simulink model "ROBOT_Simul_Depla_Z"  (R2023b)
settings: Solver=ode15s  StartTime=0.0  StopTime=0.2  RelTol=1e-3  EnableMultiTasking=on
undefined symbols (not defined in the file): BATI1_Défaut_sldprt, BATI2_Défaut_sldprt, BATI3_Défaut_sldprt, deg, kg, m, mm, N, rad, s, STL, X, Y, Z
libraries: sm_lib x139, fl_lib x42, nesl_utility x19, slpidlib x3
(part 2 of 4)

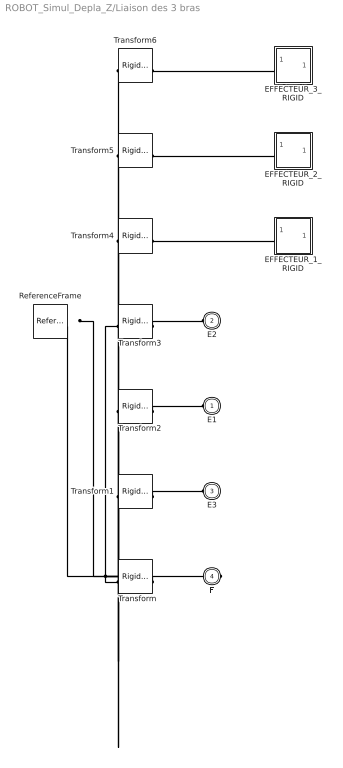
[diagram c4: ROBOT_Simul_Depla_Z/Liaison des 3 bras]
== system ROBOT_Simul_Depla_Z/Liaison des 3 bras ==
  EFFECTEUR_1_RIGID : Subsystem
  EFFECTEUR_2_RIGID : Subsystem
  EFFECTEUR_3_RIGID : Subsystem
  ReferenceFrame : sm_lib/Frames and Transforms/Reference Frame
  Transform : sm_lib/Frames and Transforms/Rigid Transform  TranslationMethod=Cartesian  TranslationStandardOffset=0  TranslationStandardOffsetUnits=mm  TranslationStandardAxis=+Z  TranslationCartesianOffset=[0 0 -32.350000000009082]  TranslationCartesianOffsetUnits=mm  TranslationROffset=0  TranslationROffsetUnits=m  TranslationZOffset=0  TranslationZOffsetUnits=m  TranslationThetaOffset=0  TranslationThetaOffsetUnits=deg  RotationMethod=ArbitraryAxis  RotationAngleUnits=rad  RotationStandardAxis=+Z  RotationAngle=3.1415926535897931  RotationArbitraryAxis=[1 0 0]  FollAlignAxisA=+X  BaseAlignAxisA=+Y  FollAlignAxisB=+Y  BaseAlignAxisB=+Z  RotationSequenceAxes=FollowerAxes  RotationSequence=XYX  RotationSequenceAngles=[0 0 0]  RotationSequenceAnglesUnits=deg  RotationMatrix=[1 0 0; 0 1 0; 0 0 1]  Quaternion=[1 0 0 0]
  Transform1 : sm_lib/Frames and Transforms/Rigid Transform  TranslationMethod=Cartesian  TranslationStandardOffset=0  TranslationStandardOffsetUnits=mm  TranslationStandardAxis=+Z  TranslationCartesianOffset=[-19.120111238677367 -12.995546039657871 14.999999999991132]  TranslationCartesianOffsetUnits=mm  TranslationROffset=0  TranslationROffsetUnits=m  TranslationZOffset=0  TranslationZOffsetUnits=m  TranslationThetaOffset=0  TranslationThetaOffsetUnits=deg  RotationMethod=ArbitraryAxis  RotationAngleUnits=rad  RotationStandardAxis=+Z  RotationAngle=2.4188584057763762  RotationArbitraryAxis=[-0.65465367070797653 -0.37796447300922748 -0.65465367070797764]  FollAlignAxisA=+X  BaseAlignAxisA=+Y  FollAlignAxisB=+Y  BaseAlignAxisB=+Z  RotationSequenceAxes=FollowerAxes  RotationSequence=XYX  RotationSequenceAngles=[0 0 0]  RotationSequenceAnglesUnits=deg  RotationMatrix=[1 0 0; 0 1 0; 0 0 1]  Quaternion=[1 0 0 0]
  Transform2 : sm_lib/Frames and Transforms/Rigid Transform  TranslationMethod=Cartesian  TranslationStandardOffset=0  TranslationStandardOffsetUnits=mm  TranslationStandardAxis=+Z  TranslationCartesianOffset=[2.6286000672859817 43.296105206329507 14.999999999990896]  TranslationCartesianOffsetUnits=mm  TranslationROffset=0  TranslationROffsetUnits=m  TranslationZOffset=0  TranslationZOffsetUnits=m  TranslationThetaOffset=0  TranslationThetaOffsetUnits=deg  RotationMethod=ArbitraryAxis  RotationAngleUnits=rad  RotationStandardAxis=+Z  RotationAngle=2.4188584057763851  RotationArbitraryAxis=[0.65465367070797842 -0.37796447300922287 0.65465367070797842]  FollAlignAxisA=+X  BaseAlignAxisA=+Y  FollAlignAxisB=+Y  BaseAlignAxisB=+Z  RotationSequenceAxes=FollowerAxes  RotationSequence=XYX  RotationSequenceAngles=[0 0 0]  RotationSequenceAnglesUnits=deg  RotationMatrix=[1 0 0; 0 1 0; 0 0 1]  Quaternion=[1 0 0 0]
  Transform3 : sm_lib/Frames and Transforms/Rigid Transform  TranslationMethod=Cartesian  TranslationStandardOffset=0  TranslationStandardOffsetUnits=mm  TranslationStandardAxis=+Z  TranslationCartesianOffset=[43.004244414304381 -8.0147839261255491 14.99999999999091]  TranslationCartesianOffsetUnits=mm  TranslationROffset=0  TranslationROffsetUnits=m  TranslationZOffset=0  TranslationZOffsetUnits=m  TranslationThetaOffset=0  TranslationThetaOffsetUnits=deg  RotationMethod=ArbitraryAxis  RotationAngleUnits=rad  RotationStandardAxis=+Z  RotationAngle=2.0943951023931993  RotationArbitraryAxis=[-0.57735026918962318 -0.57735026918962706 0.57735026918962695]  FollAlignAxisA=+X  BaseAlignAxisA=+Y  FollAlignAxisB=+Y  BaseAlignAxisB=+Z  RotationSequenceAxes=FollowerAxes  RotationSequence=XYX  RotationSequenceAngles=[0 0 0]  RotationSequenceAnglesUnits=deg  RotationMatrix=[1 0 0; 0 1 0; 0 0 1]  Quaternion=[1 0 0 0]
  Transform4 : sm_lib/Frames and Transforms/Rigid Transform  TranslationMethod=Cartesian  TranslationStandardOffset=0  TranslationStandardOffsetUnits=mm  TranslationStandardAxis=+Z  TranslationCartesianOffset=[8.0042444143042797 5.9852160738742057 -9.0899510141184692e-12]  TranslationCartesianOffsetUnits=mm  TranslationROffset=0  TranslationROffsetUnits=m  TranslationZOffset=0  TranslationZOffsetUnits=m  TranslationThetaOffset=0  TranslationThetaOffsetUnits=deg  RotationMethod=None  RotationAngleUnits=deg  RotationStandardAxis=+Z  RotationAngle=0  RotationArbitraryAxis=[0 0 1]  FollAlignAxisA=+X  BaseAlignAxisA=+Y  FollAlignAxisB=+Y  BaseAlignAxisB=+Z  RotationSequenceAxes=FollowerAxes  RotationSequence=XYX  RotationSequenceAngles=[0 0 0]  RotationSequenceAnglesUnits=deg  RotationMatrix=[1 0 0; 0 1 0; 0 0 1]  Quaternion=[1 0 0 0]
  Transform5 : sm_lib/Frames and Transforms/Rigid Transform  TranslationMethod=Cartesian  TranslationStandardOffset=0  TranslationStandardOffsetUnits=mm  TranslationStandardAxis=+Z  TranslationCartesianOffset=[8.0042444143042797 5.9852160738742057 -9.0899510141184692e-12]  TranslationCartesianOffsetUnits=mm  TranslationROffset=0  TranslationROffsetUnits=m  TranslationZOffset=0  TranslationZOffsetUnits=m  TranslationThetaOffset=0  TranslationThetaOffsetUnits=deg  RotationMethod=ArbitraryAxis  RotationAngleUnits=rad  RotationStandardAxis=+Z  RotationAngle=2.0943951023932001  RotationArbitraryAxis=[0 0 1]  FollAlignAxisA=+X  BaseAlignAxisA=+Y  FollAlignAxisB=+Y  BaseAlignAxisB=+Z  RotationSequenceAxes=FollowerAxes  RotationSequence=XYX  RotationSequenceAngles=[0 0 0]  RotationSequenceAnglesUnits=deg  RotationMatrix=[1 0 0; 0 1 0; 0 0 1]  Quaternion=[1 0 0 0]
  Transform6 : sm_lib/Frames and Transforms/Rigid Transform  TranslationMethod=Cartesian  TranslationStandardOffset=0  TranslationStandardOffsetUnits=mm  TranslationStandardAxis=+Z  TranslationCartesianOffset=[8.0042444143042797 5.9852160738742057 -9.0899510141184692e-12]  TranslationCartesianOffsetUnits=mm  TranslationROffset=0  TranslationROffsetUnits=m  TranslationZOffset=0  TranslationZOffsetUnits=m  TranslationThetaOffset=0  TranslationThetaOffsetUnits=deg  RotationMethod=ArbitraryAxis  RotationAngleUnits=rad  RotationStandardAxis=+Z  RotationAngle=2.0943951023931859  RotationArbitraryAxis=[-0 -0 -1]  FollAlignAxisA=+X  BaseAlignAxisA=+Y  FollAlignAxisB=+Y  BaseAlignAxisB=+Z  RotationSequenceAxes=FollowerAxes  RotationSequence=XYX  RotationSequenceAngles=[0 0 0]  RotationSequenceAnglesUnits=deg  RotationMatrix=[1 0 0; 0 1 0; 0 0 1]  Quaternion=[1 0 0 0]
  E1 : PMIOPort  Side=Left
  E2 : PMIOPort  Port=2  Side=Left
  E3 : PMIOPort  Port=3  Side=Left
  F : PMIOPort  Port=4  Side=Right
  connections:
  Transform/LConn1 -- ReferenceFrame/RConn1 -- Transform1/LConn1 -- Transform2/LConn1 -- Transform3/LConn1 -- Transform4/LConn1 -- Transform5/LConn1 -- Transform6/LConn1
  Transform/RConn1 -- F/RConn1
  Transform1/RConn1 -- E3/RConn1
  Transform2/RConn1 -- E1/RConn1
  Transform3/RConn1 -- E2/RConn1
  EFFECTEUR_1_RIGID/LConn1 -- Transform4/RConn1
  EFFECTEUR_2_RIGID/LConn1 -- Transform5/RConn1
  EFFECTEUR_3_RIGID/LConn1 -- Transform6/RConn1

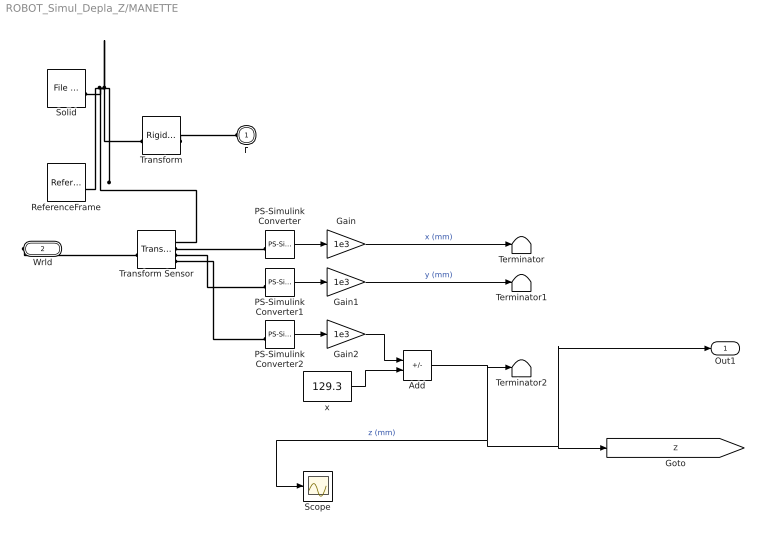
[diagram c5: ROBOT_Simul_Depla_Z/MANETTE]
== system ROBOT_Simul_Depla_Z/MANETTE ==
  Add : Sum  Inputs=+-
  Gain : Gain  Gain=1e3
  Gain1 : Gain  Gain=1e3
  Gain2 : Gain  Gain=1e3
  PS-Simulink Converter : nesl_utility/PS-Simulink Converter  PhysicalDomain=network_engine_domain  SubClassName=ps_output  LeftPortType=input  RightPortType=output  PseudoPeriodic=off  Frequencies=[]  VectorFormat=1-D array  Unit=1  AffineConversion=off
  PS-Simulink Converter1 : nesl_utility/PS-Simulink Converter  PhysicalDomain=network_engine_domain  SubClassName=ps_output  LeftPortType=input  RightPortType=output  PseudoPeriodic=off  Frequencies=[]  VectorFormat=1-D array  Unit=1  AffineConversion=off
  PS-Simulink Converter2 : nesl_utility/PS-Simulink Converter  PhysicalDomain=network_engine_domain  SubClassName=ps_output  LeftPortType=input  RightPortType=output  PseudoPeriodic=off  Frequencies=[]  VectorFormat=1-D array  Unit=1  AffineConversion=off
  ReferenceFrame : sm_lib/Frames and Transforms/Reference Frame
  Scope : Scope
  Solid : sm_lib/Body Elements/File Solid  ExtGeomFileName=\STL\MANETTE_Défaut_sldprt.STL  UnitType=Custom  ExtGeomFileUnits=mm  StepReaderType=HEX  ExportConvexHullGeometry=off  InertiaType=Custom  Mass=0.040615337241087436  MassUnits=kg  CenterOfMass=[0 0.040047984959972249 0]  CenterOfMassUnits=mm  MomentsOfInertia=[8.2576276174464649 8.2126567442848692 8.2576263457676724]  MomentsOfInertiaUnits=kg*mm^2  ProductsOfInertia=[0 0 0]  ProductsOfInertiaUnits=kg*mm^2  BasedOnType=Density  Density=1000  DensityUnits=kg/(m^3)  DoExposeReferenceFrame=on  SerializedFrames=<Frames/>  GraphicType=FromGeometry  MarkerShape=Sphere  MarkerSize=10  MarkerSizeUnits=m  GraphicVisPropType=SimpleVisualProperties  GraphicDiffuseColor=[0.69803921568627447 0.69803921568627447 0.69803921568627447]  GraphicSpecularColor=[0.5 0.5 0.5 1.0]  GraphicAmbientColor=[0.15 0.15 0.15 1.0]  GraphicEmissiveColor=[0.0 0.0 0.0 1.0]  GraphicShininess=75  GraphicOpacity=1
  Terminator : Terminator
  Terminator1 : Terminator
  Terminator2 : Terminator
  Transform : sm_lib/Frames and Transforms/Rigid Transform  TranslationMethod=Cartesian  TranslationStandardOffset=0  TranslationStandardOffsetUnits=mm  TranslationStandardAxis=+Z  TranslationCartesianOffset=[-8.0042444143042815 2.4868995751603507e-14 5.9852160738742031]  TranslationCartesianOffsetUnits=mm  TranslationROffset=0  TranslationROffsetUnits=m  TranslationZOffset=0  TranslationZOffsetUnits=m  TranslationThetaOffset=0  TranslationThetaOffsetUnits=deg  RotationMethod=ArbitraryAxis  RotationAngleUnits=rad  RotationStandardAxis=+Z  RotationAngle=1.570796326794897  RotationArbitraryAxis=[1 -1.5700924586837747e-16 -7.5435830438090697e-17]  FollAlignAxisA=+X  BaseAlignAxisA=+Y  FollAlignAxisB=+Y  BaseAlignAxisB=+Z  RotationSequenceAxes=FollowerAxes  RotationSequence=XYX  RotationSequenceAngles=[0 0 0]  RotationSequenceAnglesUnits=deg  RotationMatrix=[1 0 0; 0 1 0; 0 0 1]  Quaternion=[1 0 0 0]
  Transform Sensor : sm_lib/Frames and Transforms/Transform Sensor  MeasurementFrame=World  RotationSequence=XYX  SenseAngle=off  SenseAxis=off  SenseQ=off  SenseR=off  SenseRotationSequence=off  SenseOmegaX=off  SenseOmegaY=off  SenseOmegaZ=off  SenseOmega=off  SenseQDot=off  SenseRDot=off  SenseRotationSequenceDot=off  SenseAlphaX=off  SenseAlphaY=off  SenseAlphaZ=off  SenseAlpha=off  SenseQDDot=off  SenseRDDot=off  SenseX=on  SenseY=on  SenseZ=on  SenseXYZ=off  SenseRad=off  SenseAzim=off  SenseDist=off  SenseInc=off  SenseXDot=off  SenseYDot=off  SenseZDot=off  SenseXYZDot=off  SenseRadDot=off  SenseAzimDot=off  SenseDistDot=off  SenseIncDot=off  SenseXDDot=off  SenseYDDot=off  SenseZDDot=off  SenseXYZDDot=off  SenseRadDDot=off  SenseAzimDDot=off  SenseDistDDot=off  SenseIncDDot=off
  x : Constant  Value=129.3
  F : PMIOPort  Side=Left
  Wrld : PMIOPort  Port=2  Side=Right
  Out1 : Outport  VectorParamsAs1DForOutWhenUnconnected=off
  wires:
  Gain1/1 -> Terminator1/1  "y (mm)"
  PS-Simulink Converter2/1 -> Gain2/1
  x/1 -> Add/2
  Add/1 -> Scope/1, Out1/1, [Z], Terminator2/1  "z (mm)"
  PS-Simulink Converter1/1 -> Gain1/1
  Gain2/1 -> Add/1
  PS-Simulink Converter/1 -> Gain/1
  Gain/1 -> Terminator/1  "x (mm)"
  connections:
  Solid/RConn1 -- ReferenceFrame/RConn1 -- Transform Sensor/RConn1 -- Transform/LConn1
  Transform/RConn1 -- F/RConn1
  PS-Simulink Converter2/LConn1 -- Transform Sensor/RConn4
  Transform Sensor/RConn3 -- PS-Simulink Converter1/LConn1
  Transform Sensor/RConn2 -- PS-Simulink Converter/LConn1
  Wrld/RConn1 -- Transform Sensor/LConn1

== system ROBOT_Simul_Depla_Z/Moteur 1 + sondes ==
  In1 : Inport
  Moteur à courant continu1 : Subsystem
  Reference electrique : fl_lib/Electrical/Electrical Elements/Electrical Reference
  Simulink-PS Converter1 : nesl_utility/Simulink-PS Converter  PhysicalDomain=network_engine_domain  SubClassName=ps_input  LeftPortType=input  RightPortType=output  PseudoPeriodic=off  Frequencies=[]  NoiseDistribution=none  NoiseParameters=[]  Unit=V  AffineConversion=off  FilteringAndDerivatives=zero  SimscapeFilterOrder=2  InputFilterTimeConstant=1e-4  UdotUserProvided=1
  Sondes électriques1 : Subsystem
  Source de tension controlée1 : fl_lib/Electrical/Electrical Sources/Controlled Voltage Source
  Conn1 : PMIOPort  Side=Right
  Conn2 : PMIOPort  Port=2  Side=Right
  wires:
  In1/1 -> Simulink-PS Converter1/1
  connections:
  Conn2/RConn1 -- Moteur à courant continu1/RConn2
  Conn1/RConn1 -- Moteur à courant continu1/RConn1
  Source de tension controlée1/LConn1 -- Sondes électriques1/LConn1
  Simulink-PS Converter1/RConn1 -- Source de tension controlée1/RConn1
  Sondes électriques1/RConn2 -- Source de tension controlée1/RConn2 -- Reference electrique/LConn1 -- Moteur à courant continu1/LConn2
  Sondes électriques1/RConn1 -- Moteur à courant continu1/LConn1

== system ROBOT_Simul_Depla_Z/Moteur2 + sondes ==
  In1 : Inport
  Moteur à courant continu2 : Subsystem
  Reference electrique : fl_lib/Electrical/Electrical Elements/Electrical Reference
  Simulink-PS Converter1 : nesl_utility/Simulink-PS Converter  PhysicalDomain=network_engine_domain  SubClassName=ps_input  LeftPortType=input  RightPortType=output  PseudoPeriodic=off  Frequencies=[]  NoiseDistribution=none  NoiseParameters=[]  Unit=V  AffineConversion=off  FilteringAndDerivatives=zero  SimscapeFilterOrder=2  InputFilterTimeConstant=1e-4  UdotUserProvided=1
  Sondes électriques : Subsystem
  Source de tension controlée : fl_lib/Electrical/Electrical Sources/Controlled Voltage Source
  Conn1 : PMIOPort  Side=Right
  Conn2 : PMIOPort  Port=2  Side=Right
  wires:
  In1/1 -> Simulink-PS Converter1/1
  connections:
  Sondes électriques/RConn1 -- Moteur à courant continu2/LConn1
  Source de tension controlée/RConn2 -- Reference electrique/LConn1 -- Sondes électriques/RConn2 -- Moteur à courant continu2/LConn2
  Simulink-PS Converter1/RConn1 -- Source de tension controlée/RConn1
  Source de tension controlée/LConn1 -- Sondes électriques/LConn1
  Conn1/RConn1 -- Moteur à courant continu2/RConn1
  Conn2/RConn1 -- Moteur à courant continu2/RConn2

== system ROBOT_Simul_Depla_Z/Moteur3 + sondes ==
  In1 : Inport
  Moteur à courant continu3 : Subsystem
  Reference electrique : fl_lib/Electrical/Electrical Elements/Electrical Reference
  Simulink-PS Converter1 : nesl_utility/Simulink-PS Converter  PhysicalDomain=network_engine_domain  SubClassName=ps_input  LeftPortType=input  RightPortType=output  PseudoPeriodic=off  Frequencies=[]  NoiseDistribution=none  NoiseParameters=[]  Unit=V  AffineConversion=off  FilteringAndDerivatives=zero  SimscapeFilterOrder=2  InputFilterTimeConstant=1e-4  UdotUserProvided=1
  Sondes électriques3 : Subsystem
  Source de tension controlée3 : fl_lib/Electrical/Electrical Sources/Controlled Voltage Source
  Conn1 : PMIOPort  Side=Right
  Conn2 : PMIOPort  Port=2  Side=Right
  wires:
  In1/1 -> Simulink-PS Converter1/1
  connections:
  Sondes électriques3/RConn1 -- Moteur à courant continu3/LConn1
  Moteur à courant continu3/LConn2 -- Reference electrique/LConn1 -- Source de tension controlée3/RConn2 -- Sondes électriques3/RConn2
  Simulink-PS Converter1/RConn1 -- Source de tension controlée3/RConn1
  Source de tension controlée3/LConn1 -- Sondes électriques3/LConn1
  Conn1/RConn1 -- Moteur à courant continu3/RConn1
  Conn2/RConn1 -- Moteur à courant continu3/RConn2

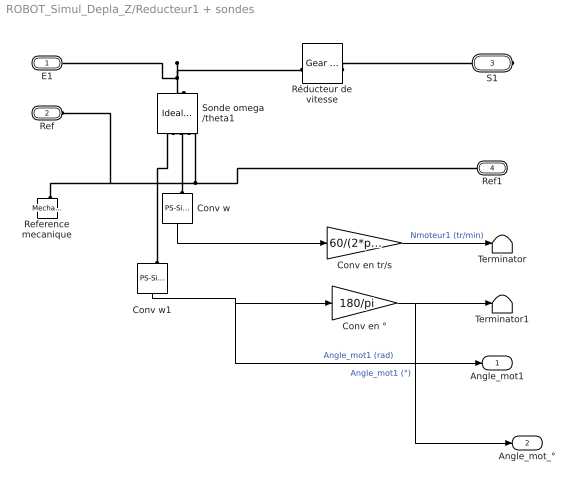
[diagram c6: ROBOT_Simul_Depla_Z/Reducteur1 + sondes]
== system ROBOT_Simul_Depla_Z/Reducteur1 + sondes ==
  Conv en tr/s : Gain  Gain=60/(2*pi)
  Conv en ° : Gain  Gain=180/pi
  Conv w : nesl_utility/PS-Simulink Converter  PhysicalDomain=network_engine_domain  SubClassName=ps_output  LeftPortType=input  RightPortType=output  PseudoPeriodic=off  Frequencies=[]  VectorFormat=1-D array  Unit=1  AffineConversion=off
  Conv w1 : nesl_utility/PS-Simulink Converter  PhysicalDomain=network_engine_domain  SubClassName=ps_output  LeftPortType=input  RightPortType=output  PseudoPeriodic=off  Frequencies=[]  VectorFormat=1-D array  Unit=1  AffineConversion=off
  Reference mecanique : fl_lib/Mechanical/Rotational Elements/Mechanical Rotational Reference
  Réducteur de vitesse : fl_lib/Mechanical/Mechanisms/Gear Box  ratio=7.627  t_in_specify=off  t_in_priority=None  t_in=0 N*m  t_in_nominal_specify=off  t_in_nominal_unit=N*m  t_in_nominal_value=1  t_out_specify=off  t_out_priority=None  t_out=0 N*m  t_out_nominal_specify=off  t_out_nominal_unit=N*m  t_out_nominal_value=1
  Sonde omega /theta1 : fl_lib/Mechanical/Mechanical Sensors/Ideal Rotational Motion Sensor  reference=foundation.enum.MeasurementReference.difference  acceleration_port=false  velocity_port=true  position_port=true  wrap_angle=false  offset=0 rad
  Terminator : Terminator
  Terminator1 : Terminator
  E1 : PMIOPort  Side=Left
  Ref : PMIOPort  Port=2  Side=Left
  S1 : PMIOPort  Port=3  Side=Right
  Ref1 : PMIOPort  Port=4  Side=Right
  Angle_mot1 : Outport  VectorParamsAs1DForOutWhenUnconnected=off
  Angle_mot_° : Outport  Port=2  VectorParamsAs1DForOutWhenUnconnected=off
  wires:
  Conv w1/1 -> Angle_mot1/1, Conv en °/1  "Angle_mot1 (rad)"
  Conv en °/1 -> Angle_mot_°/1, Terminator1/1  "Angle_mot1 (°)"
  Conv w/1 -> Conv en tr/s/1
  Conv en tr/s/1 -> Terminator/1  "Nmoteur1 (tr/min)"
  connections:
  Sonde omega /theta1/LConn1 -- E1/RConn1 -- Réducteur de vitesse/LConn1
  Reference mecanique/LConn1 -- Ref/RConn1 -- Sonde omega /theta1/RConn1 -- Ref1/RConn1
  Conv w/LConn1 -- Sonde omega /theta1/RConn2
  Conv w1/LConn1 -- Sonde omega /theta1/RConn3
  Réducteur de vitesse/RConn1 -- S1/RConn1

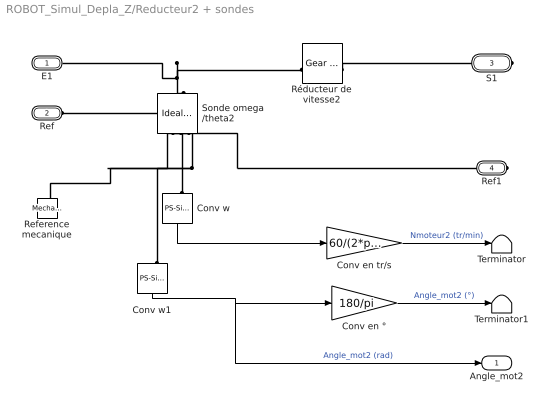
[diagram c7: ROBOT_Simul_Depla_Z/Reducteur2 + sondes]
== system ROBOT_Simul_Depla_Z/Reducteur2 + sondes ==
  Conv en tr/s : Gain  Gain=60/(2*pi)
  Conv en ° : Gain  Gain=180/pi
  Conv w : nesl_utility/PS-Simulink Converter  PhysicalDomain=network_engine_domain  SubClassName=ps_output  LeftPortType=input  RightPortType=output  PseudoPeriodic=off  Frequencies=[]  VectorFormat=1-D array  Unit=1  AffineConversion=off
  Conv w1 : nesl_utility/PS-Simulink Converter  PhysicalDomain=network_engine_domain  SubClassName=ps_output  LeftPortType=input  RightPortType=output  PseudoPeriodic=off  Frequencies=[]  VectorFormat=1-D array  Unit=1  AffineConversion=off
  Reference mecanique : fl_lib/Mechanical/Rotational Elements/Mechanical Rotational Reference
  Réducteur de vitesse2 : fl_lib/Mechanical/Mechanisms/Gear Box  ratio=7.627  t_in_specify=off  t_in_priority=None  t_in=0 N*m  t_in_nominal_specify=off  t_in_nominal_unit=N*m  t_in_nominal_value=1  t_out_specify=off  t_out_priority=None  t_out=0 N*m  t_out_nominal_specify=off  t_out_nominal_unit=N*m  t_out_nominal_value=1
  Sonde omega /theta2 : fl_lib/Mechanical/Mechanical Sensors/Ideal Rotational Motion Sensor  reference=foundation.enum.MeasurementReference.difference  acceleration_port=false  velocity_port=true  position_port=true  wrap_angle=false  offset=0 rad
  Terminator : Terminator
  Terminator1 : Terminator
  E1 : PMIOPort  Side=Left
  Ref : PMIOPort  Port=2  Side=Left
  S1 : PMIOPort  Port=3  Side=Right
  Ref1 : PMIOPort  Port=4  Side=Right
  Angle_mot2 : Outport  VectorParamsAs1DForOutWhenUnconnected=off
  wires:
  Conv w1/1 -> Angle_mot2/1, Conv en °/1  "Angle_mot2 (rad)"
  Conv en °/1 -> Terminator1/1  "Angle_mot2 (°)"
  Conv w/1 -> Conv en tr/s/1
  Conv en tr/s/1 -> Terminator/1  "Nmoteur2 (tr/min)"
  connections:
  Sonde omega /theta2/LConn1 -- E1/RConn1 -- Réducteur de vitesse2/LConn1
  Ref1/RConn1 -- Sonde omega /theta2/RConn1 -- Reference mecanique/LConn1 -- Ref/RConn1
  Conv w1/LConn1 -- Sonde omega /theta2/RConn3
  Conv w/LConn1 -- Sonde omega /theta2/RConn2
  Réducteur de vitesse2/RConn1 -- S1/RConn1

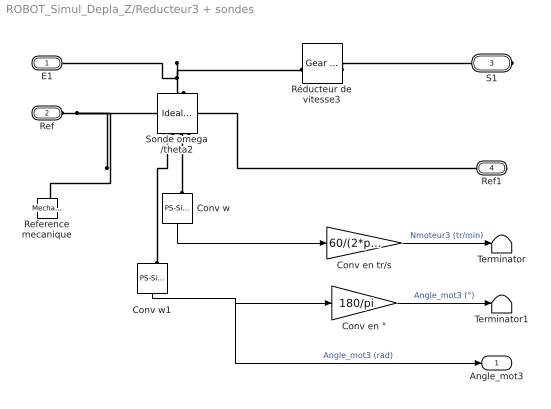
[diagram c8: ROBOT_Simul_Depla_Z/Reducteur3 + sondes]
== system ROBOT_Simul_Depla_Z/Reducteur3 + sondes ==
  Conv en tr/s : Gain  Gain=60/(2*pi)
  Conv en ° : Gain  Gain=180/pi
  Conv w : nesl_utility/PS-Simulink Converter  PhysicalDomain=network_engine_domain  SubClassName=ps_output  LeftPortType=input  RightPortType=output  PseudoPeriodic=off  Frequencies=[]  VectorFormat=1-D array  Unit=1  AffineConversion=off
  Conv w1 : nesl_utility/PS-Simulink Converter  PhysicalDomain=network_engine_domain  SubClassName=ps_output  LeftPortType=input  RightPortType=output  PseudoPeriodic=off  Frequencies=[]  VectorFormat=1-D array  Unit=1  AffineConversion=off
  Reference mecanique : fl_lib/Mechanical/Rotational Elements/Mechanical Rotational Reference
  Réducteur de vitesse3 : fl_lib/Mechanical/Mechanisms/Gear Box  ratio=-7.627  t_in_specify=off  t_in_priority=None  t_in=0 N*m  t_in_nominal_specify=off  t_in_nominal_unit=N*m  t_in_nominal_value=1  t_out_specify=off  t_out_priority=None  t_out=0 N*m  t_out_nominal_specify=off  t_out_nominal_unit=N*m  t_out_nominal_value=1
  Sonde omega /theta2 : fl_lib/Mechanical/Mechanical Sensors/Ideal Rotational Motion Sensor  reference=foundation.enum.MeasurementReference.difference  acceleration_port=false  velocity_port=true  position_port=true  wrap_angle=false  offset=0 rad
  Terminator : Terminator
  Terminator1 : Terminator
  E1 : PMIOPort  Side=Left
  Ref : PMIOPort  Port=2  Side=Left
  S1 : PMIOPort  Port=3  Side=Right
  Ref1 : PMIOPort  Port=4  Side=Right
  Angle_mot3 : Outport  VectorParamsAs1DForOutWhenUnconnected=off
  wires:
  Conv w1/1 -> Angle_mot3/1, Conv en °/1  "Angle_mot3 (rad)"
  Conv en °/1 -> Terminator1/1  "Angle_mot3 (°)"
  Conv w/1 -> Conv en tr/s/1
  Conv en tr/s/1 -> Terminator/1  "Nmoteur3 (tr/min)"
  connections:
  Sonde omega /theta2/LConn1 -- E1/RConn1 -- Réducteur de vitesse3/LConn1
  Ref/RConn1 -- Reference mecanique/LConn1 -- Sonde omega /theta2/RConn1 -- Ref1/RConn1
  Conv w1/LConn1 -- Sonde omega /theta2/RConn3
  Réducteur de vitesse3/RConn1 -- S1/RConn1
  Conv w/LConn1 -- Sonde omega /theta2/RConn2

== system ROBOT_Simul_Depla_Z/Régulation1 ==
  In1 : Inport
  In2 : Inport  Port=2
  Add : Sum  Inputs=-+
  PID Controller : slpidlib/PID Controller  Controller=PD  Form=Parallel  TimeDomain=Continuous-time  UseExternalTs=off  SampleTime=1  IntegratorMethod=Forward Euler  FilterMethod=Forward Euler  ControllerParametersSource=internal  P=200  I=30  UseKiTs=off  D=4  N=900  UseFilter=on  TunerSelectOption=Transfer Function Based (PID Tuner App)  ZeroCross=off  InitialConditionSource=internal  InitialConditionForIntegrator=0  InitialConditionForFilter=0  DifferentiatorICPrevScaledInput=0  ExternalReset=none  TrackingMode=off  Kt=1  LimitOutput=on  SatLimitsSource=internal  UpperSaturationLimit=30  LowerSaturationLimit=-30  LinearizeAsGain=off  AntiWindupMode=none  Kb=1  LimitIntegrator=off  UpperIntegratorSaturationLimit=inf  LowerIntegratorSaturationLimit=-inf  POutMin=[]  POutMax=[]  IOutMin=[]  IOutMax=[]  DOutMin=[]  DOutMax=[]  NOutMin=[]  NOutMax=[]  SumOutMin=[]  SumOutMax=[]  SaturationOutMin=[]  SaturationOutMax=[]  PParamMin=[]  PParamMax=[]  IParamMin=[]  IParamMax=[]  DParamMin=[]  DParamMax=[]  NParamMin=[]  NParamMax=[]  KbParamMin=[]  KbParamMax=[]  KtParamMin=[]  KtParamMax=[]  KbOutMin=[]  KbOutMax=[]  KtOutMin=[]  KtOutMax=[]  IntegratorOutMin=[]  IntegratorOutMax=[]  FilterOutMin=[]  FilterOutMax=[]  SumI1OutMin=[]  SumI1OutMax=[]  SumI2OutMin=[]  SumI2OutMax=[]  SumI3OutMin=[]  SumI3OutMax=[]  SumI4OutMin=[]  SumI4OutMax=[]  SumDOutMin=[]  SumDOutMax=[]  DifferentiatorOutMin=[]  DifferentiatorOutMax=[]  FilterDiffOutCoefMin=[]  FilterDiffOutCoefMax=[]  ReciprocalOutMin=[]  ReciprocalOutMax=[]  SumDenOutMin=[]  SumDenOutMax=[]  SumNumOutMin=[]  SumNumOutMax=[]  DivideOutMin=[]  DivideOutMax=[]  UdiffTsProdOutMin=[]  UdiffTsProdOutMax=[]  NTsProdOutMin=[]  NTsProdOutMax=[]  UintegralTsProdOutMin=[]  UintegralTsProdOutMax=[]  UngainTsProdOutMin=[]  UngainTsProdOutMax=[]  ClampingZeroOutDataTypeStr=Inherit: Inherit via back propagation  ClampingZeroOutMin=[]  ClampingZeroOutMax=[]  FilterDenConstantOutDataTypeStr=Inherit: Inherit via back propagation  FilterDenConstantOutMin=[]  FilterDenConstantOutMax=[]  PCopyOutDataTypeStr=Inherit: Inherit via back propagation  PCopyOutMin=[]  PCopyOutMax=[]  NCopyOutDataTypeStr=Inherit: Inherit via back propagation  NCopyOutMin=[]  NCopyOutMax=[]  IntegratorContinuousStateAttributes=''  IntegratorStateMustResolveToSignalObject=off  IntegratorRTWStateStorageClass=Auto  FilterContinuousStateAttributes=''  FilterStateMustResolveToSignalObject=off  FilterRTWStateStorageClass=Auto  ParallelPVariant=InternalParameters  IdealPVariant=Disabled  IVariant=Disabled  DVariant=InternalParameters  IntegratorVariant=Disabled  SatVariant=Enabled  AWVariant=Disabled  PCopyVariant=Disabled  TRVariant=Disabled  FdbkBlocksVariant=Forward  IdealPFdbkVariant=Disabled  SatFdbkVariant=Disabled  DerivativeFilterVariant=ContFilter  NVariant=InternalParameters  NCopyVariant=Disabled  FilterICVariant=InternalICsFilter  IntegratorICVariant=Disabled  ExternalResetVariant=Disabled  TRSumVariant=Passthrough  SumFdbkVariant=Disabled  SumVariant=Sum_PD  TsampFilterVariant=InternalTs  TsampNgainVariant=Passthrough  TsampIntegralVariant=Disabled_SignalSpec  ExternalSaturationOutDataTypeStr=Inherit: Same as second input
  Out1 : Outport  VectorParamsAs1DForOutWhenUnconnected=off
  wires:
  In1/1 -> Add/1
  In2/1 -> Add/2
  PID Controller/1 -> Out1/1
  Add/1 -> PID Controller/1

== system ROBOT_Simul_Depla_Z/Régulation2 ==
  In1 : Inport
  In2 : Inport  Port=2
  Add : Sum  Inputs=-+
  PID Controller : slpidlib/PID Controller  Controller=PD  Form=Parallel  TimeDomain=Continuous-time  UseExternalTs=off  SampleTime=1  IntegratorMethod=Forward Euler  FilterMethod=Forward Euler  ControllerParametersSource=internal  P=200  I=30  UseKiTs=off  D=4  N=900  UseFilter=on  TunerSelectOption=Transfer Function Based (PID Tuner App)  ZeroCross=off  InitialConditionSource=internal  InitialConditionForIntegrator=0  InitialConditionForFilter=0  DifferentiatorICPrevScaledInput=0  ExternalReset=none  TrackingMode=off  Kt=1  LimitOutput=on  SatLimitsSource=internal  UpperSaturationLimit=30  LowerSaturationLimit=-30  LinearizeAsGain=off  AntiWindupMode=none  Kb=1  LimitIntegrator=off  UpperIntegratorSaturationLimit=inf  LowerIntegratorSaturationLimit=-inf  POutMin=[]  POutMax=[]  IOutMin=[]  IOutMax=[]  DOutMin=[]  DOutMax=[]  NOutMin=[]  NOutMax=[]  SumOutMin=[]  SumOutMax=[]  SaturationOutMin=[]  SaturationOutMax=[]  PParamMin=[]  PParamMax=[]  IParamMin=[]  IParamMax=[]  DParamMin=[]  DParamMax=[]  NParamMin=[]  NParamMax=[]  KbParamMin=[]  KbParamMax=[]  KtParamMin=[]  KtParamMax=[]  KbOutMin=[]  KbOutMax=[]  KtOutMin=[]  KtOutMax=[]  IntegratorOutMin=[]  IntegratorOutMax=[]  FilterOutMin=[]  FilterOutMax=[]  SumI1OutMin=[]  SumI1OutMax=[]  SumI2OutMin=[]  SumI2OutMax=[]  SumI3OutMin=[]  SumI3OutMax=[]  SumI4OutMin=[]  SumI4OutMax=[]  SumDOutMin=[]  SumDOutMax=[]  DifferentiatorOutMin=[]  DifferentiatorOutMax=[]  FilterDiffOutCoefMin=[]  FilterDiffOutCoefMax=[]  ReciprocalOutMin=[]  ReciprocalOutMax=[]  SumDenOutMin=[]  SumDenOutMax=[]  SumNumOutMin=[]  SumNumOutMax=[]  DivideOutMin=[]  DivideOutMax=[]  UdiffTsProdOutMin=[]  UdiffTsProdOutMax=[]  NTsProdOutMin=[]  NTsProdOutMax=[]  UintegralTsProdOutMin=[]  UintegralTsProdOutMax=[]  UngainTsProdOutMin=[]  UngainTsProdOutMax=[]  ClampingZeroOutDataTypeStr=Inherit: Inherit via back propagation  ClampingZeroOutMin=[]  ClampingZeroOutMax=[]  FilterDenConstantOutDataTypeStr=Inherit: Inherit via back propagation  FilterDenConstantOutMin=[]  FilterDenConstantOutMax=[]  PCopyOutDataTypeStr=Inherit: Inherit via back propagation  PCopyOutMin=[]  PCopyOutMax=[]  NCopyOutDataTypeStr=Inherit: Inherit via back propagation  NCopyOutMin=[]  NCopyOutMax=[]  IntegratorContinuousStateAttributes=''  IntegratorStateMustResolveToSignalObject=off  IntegratorRTWStateStorageClass=Auto  FilterContinuousStateAttributes=''  FilterStateMustResolveToSignalObject=off  FilterRTWStateStorageClass=Auto  ParallelPVariant=InternalParameters  IdealPVariant=Disabled  IVariant=Disabled  DVariant=InternalParameters  IntegratorVariant=Disabled  SatVariant=Enabled  AWVariant=Disabled  PCopyVariant=Disabled  TRVariant=Disabled  FdbkBlocksVariant=Forward  IdealPFdbkVariant=Disabled  SatFdbkVariant=Disabled  DerivativeFilterVariant=ContFilter  NVariant=InternalParameters  NCopyVariant=Disabled  FilterICVariant=InternalICsFilter  IntegratorICVariant=Disabled  ExternalResetVariant=Disabled  TRSumVariant=Passthrough  SumFdbkVariant=Disabled  SumVariant=Sum_PD  TsampFilterVariant=InternalTs  TsampNgainVariant=Passthrough  TsampIntegralVariant=Disabled_SignalSpec  ExternalSaturationOutDataTypeStr=Inherit: Same as second input
  Out1 : Outport  VectorParamsAs1DForOutWhenUnconnected=off
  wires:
  Add/1 -> PID Controller/1
  PID Controller/1 -> Out1/1
  In2/1 -> Add/2
  In1/1 -> Add/1

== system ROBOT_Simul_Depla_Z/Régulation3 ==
  note: Valeurs de base P=200 D=4 N=900 P=50 I=30 D=1 N=100
  In1 : Inport
  In2 : Inport  Port=2
  Add : Sum  Inputs=-+
  PID Controller : slpidlib/PID Controller  Controller=PD  Form=Parallel  TimeDomain=Continuous-time  UseExternalTs=off  SampleTime=1  IntegratorMethod=Forward Euler  FilterMethod=Forward Euler  ControllerParametersSource=internal  P=200  I=20  UseKiTs=off  D=4  N=900  UseFilter=on  TunerSelectOption=Transfer Function Based (PID Tuner App)  ZeroCross=off  InitialConditionSource=internal  InitialConditionForIntegrator=0  InitialConditionForFilter=0  DifferentiatorICPrevScaledInput=0  ExternalReset=none  TrackingMode=off  Kt=1  LimitOutput=on  SatLimitsSource=internal  UpperSaturationLimit=30  LowerSaturationLimit=-30  LinearizeAsGain=off  AntiWindupMode=none  Kb=1  LimitIntegrator=off  UpperIntegratorSaturationLimit=inf  LowerIntegratorSaturationLimit=-inf  POutMin=[]  POutMax=[]  IOutMin=[]  IOutMax=[]  DOutMin=[]  DOutMax=[]  NOutMin=[]  NOutMax=[]  SumOutMin=[]  SumOutMax=[]  SaturationOutMin=[]  SaturationOutMax=[]  PParamMin=[]  PParamMax=[]  IParamMin=[]  IParamMax=[]  DParamMin=[]  DParamMax=[]  NParamMin=[]  NParamMax=[]  KbParamMin=[]  KbParamMax=[]  KtParamMin=[]  KtParamMax=[]  KbOutMin=[]  KbOutMax=[]  KtOutMin=[]  KtOutMax=[]  IntegratorOutMin=[]  IntegratorOutMax=[]  FilterOutMin=[]  FilterOutMax=[]  SumI1OutMin=[]  SumI1OutMax=[]  SumI2OutMin=[]  SumI2OutMax=[]  SumI3OutMin=[]  SumI3OutMax=[]  SumI4OutMin=[]  SumI4OutMax=[]  SumDOutMin=[]  SumDOutMax=[]  DifferentiatorOutMin=[]  DifferentiatorOutMax=[]  FilterDiffOutCoefMin=[]  FilterDiffOutCoefMax=[]  ReciprocalOutMin=[]  ReciprocalOutMax=[]  SumDenOutMin=[]  SumDenOutMax=[]  SumNumOutMin=[]  SumNumOutMax=[]  DivideOutMin=[]  DivideOutMax=[]  UdiffTsProdOutMin=[]  UdiffTsProdOutMax=[]  NTsProdOutMin=[]  NTsProdOutMax=[]  UintegralTsProdOutMin=[]  UintegralTsProdOutMax=[]  UngainTsProdOutMin=[]  UngainTsProdOutMax=[]  ClampingZeroOutDataTypeStr=Inherit: Inherit via back propagation  ClampingZeroOutMin=[]  ClampingZeroOutMax=[]  FilterDenConstantOutDataTypeStr=Inherit: Inherit via back propagation  FilterDenConstantOutMin=[]  FilterDenConstantOutMax=[]  PCopyOutDataTypeStr=Inherit: Inherit via back propagation  PCopyOutMin=[]  PCopyOutMax=[]  NCopyOutDataTypeStr=Inherit: Inherit via back propagation  NCopyOutMin=[]  NCopyOutMax=[]  IntegratorContinuousStateAttributes=''  IntegratorStateMustResolveToSignalObject=off  IntegratorRTWStateStorageClass=Auto  FilterContinuousStateAttributes=''  FilterStateMustResolveToSignalObject=off  FilterRTWStateStorageClass=Auto  ParallelPVariant=InternalParameters  IdealPVariant=Disabled  IVariant=Disabled  DVariant=InternalParameters  IntegratorVariant=Disabled  SatVariant=Enabled  AWVariant=Disabled  PCopyVariant=Disabled  TRVariant=Disabled  FdbkBlocksVariant=Forward  IdealPFdbkVariant=Disabled  SatFdbkVariant=Disabled  DerivativeFilterVariant=ContFilter  NVariant=InternalParameters  NCopyVariant=Disabled  FilterICVariant=InternalICsFilter  IntegratorICVariant=Disabled  ExternalResetVariant=Disabled  TRSumVariant=Passthrough  SumFdbkVariant=Disabled  SumVariant=Sum_PD  TsampFilterVariant=InternalTs  TsampNgainVariant=Passthrough  TsampIntegralVariant=Disabled_SignalSpec  ExternalSaturationOutDataTypeStr=Inherit: Same as second input
  Out1 : Outport  VectorParamsAs1DForOutWhenUnconnected=off
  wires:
  Add/1 -> PID Controller/1
  PID Controller/1 -> Out1/1
  In2/1 -> Add/2
  In1/1 -> Add/1

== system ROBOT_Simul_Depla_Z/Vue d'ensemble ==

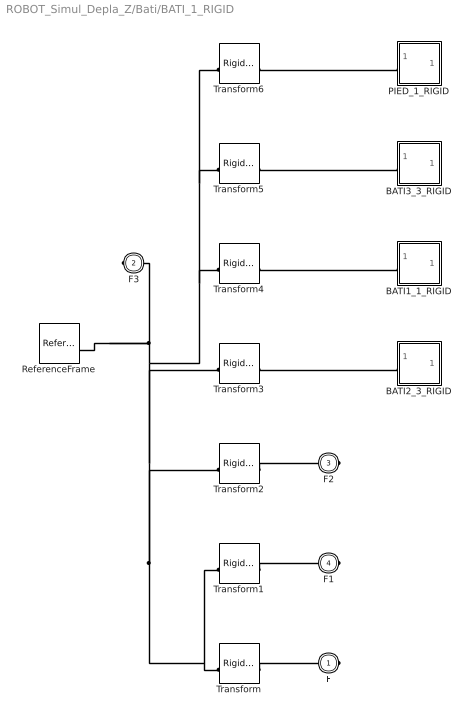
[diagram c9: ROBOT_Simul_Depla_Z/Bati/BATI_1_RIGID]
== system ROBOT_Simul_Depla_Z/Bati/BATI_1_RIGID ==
  BATI1_1_RIGID : Subsystem
  BATI2_3_RIGID : Subsystem
  BATI3_3_RIGID : Subsystem
  PIED_1_RIGID : Subsystem
  ReferenceFrame : sm_lib/Frames and Transforms/Reference Frame
  Transform : sm_lib/Frames and Transforms/Rigid Transform  TranslationMethod=Cartesian  TranslationStandardOffset=0  TranslationStandardOffsetUnits=mm  TranslationStandardAxis=+Z  TranslationCartesianOffset=[11.464585537616552 15.162590585005695 19.999999999988876]  TranslationCartesianOffsetUnits=mm  TranslationROffset=0  TranslationROffsetUnits=m  TranslationZOffset=0  TranslationZOffsetUnits=m  TranslationThetaOffset=0  TranslationThetaOffsetUnits=deg  RotationMethod=ArbitraryAxis  RotationAngleUnits=rad  RotationStandardAxis=+Z  RotationAngle=2.0943951023931953  RotationArbitraryAxis=[-0.57735026918962584 -0.57735026918962584 0.57735026918962584]  FollAlignAxisA=+X  BaseAlignAxisA=+Y  FollAlignAxisB=+Y  BaseAlignAxisB=+Z  RotationSequenceAxes=FollowerAxes  RotationSequence=XYX  RotationSequenceAngles=[0 0 0]  RotationSequenceAnglesUnits=deg  RotationMatrix=[1 0 0; 0 1 0; 0 0 1]  Quaternion=[1 0 0 0]
  Transform1 : sm_lib/Frames and Transforms/Rigid Transform  TranslationMethod=Cartesian  TranslationStandardOffset=0  TranslationStandardOffsetUnits=mm  TranslationStandardAxis=+Z  TranslationCartesianOffset=[-74.272540245284446 -12.683808110643664 19.999999999988628]  TranslationCartesianOffsetUnits=mm  TranslationROffset=0  TranslationROffsetUnits=m  TranslationZOffset=0  TranslationZOffsetUnits=m  TranslationThetaOffset=0  TranslationThetaOffsetUnits=deg  RotationMethod=ArbitraryAxis  RotationAngleUnits=rad  RotationStandardAxis=+Z  RotationAngle=2.4188584057763811  RotationArbitraryAxis=[0.65465367070797764 -0.37796447300922537 0.65465367070797764]  FollAlignAxisA=+X  BaseAlignAxisA=+Y  FollAlignAxisB=+Y  BaseAlignAxisB=+Z  RotationSequenceAxes=FollowerAxes  RotationSequence=XYX  RotationSequenceAngles=[0 0 0]  RotationSequenceAnglesUnits=deg  RotationMatrix=[1 0 0; 0 1 0; 0 0 1]  Quaternion=[1 0 0 0]
  Transform2 : sm_lib/Frames and Transforms/Rigid Transform  TranslationMethod=Cartesian  TranslationStandardOffset=0  TranslationStandardOffsetUnits=mm  TranslationStandardAxis=+Z  TranslationCartesianOffset=[-9.7882886794943111 -68.68101071934548 19.999999999988635]  TranslationCartesianOffsetUnits=mm  TranslationROffset=0  TranslationROffsetUnits=m  TranslationZOffset=0  TranslationZOffsetUnits=m  TranslationThetaOffset=0  TranslationThetaOffsetUnits=deg  RotationMethod=ArbitraryAxis  RotationAngleUnits=rad  RotationStandardAxis=+Z  RotationAngle=2.4188584057763713  RotationArbitraryAxis=[-0.65465367070797609 -0.37796447300923092 -0.65465367070797609]  FollAlignAxisA=+X  BaseAlignAxisA=+Y  FollAlignAxisB=+Y  BaseAlignAxisB=+Z  RotationSequenceAxes=FollowerAxes  RotationSequence=XYX  RotationSequenceAngles=[0 0 0]  RotationSequenceAnglesUnits=deg  RotationMatrix=[1 0 0; 0 1 0; 0 0 1]  Quaternion=[1 0 0 0]
  Transform3 : sm_lib/Frames and Transforms/Rigid Transform  TranslationMethod=Cartesian  TranslationStandardOffset=0  TranslationStandardOffsetUnits=mm  TranslationStandardAxis=+Z  TranslationCartesianOffset=[-25.865414462389737 -22.06740941499433 -1.1369377661551994e-11]  TranslationCartesianOffsetUnits=mm  TranslationROffset=0  TranslationROffsetUnits=m  TranslationZOffset=0  TranslationZOffsetUnits=m  TranslationThetaOffset=0  TranslationThetaOffsetUnits=deg  RotationMethod=None  RotationAngleUnits=deg  RotationStandardAxis=+Z  RotationAngle=0  RotationArbitraryAxis=[0 0 1]  FollAlignAxisA=+X  BaseAlignAxisA=+Y  FollAlignAxisB=+Y  BaseAlignAxisB=+Z  RotationSequenceAxes=FollowerAxes  RotationSequence=XYX  RotationSequenceAngles=[0 0 0]  RotationSequenceAnglesUnits=deg  RotationMatrix=[1 0 0; 0 1 0; 0 0 1]  Quaternion=[1 0 0 0]
  Transform4 : sm_lib/Frames and Transforms/Rigid Transform  TranslationMethod=Cartesian  TranslationStandardOffset=0  TranslationStandardOffsetUnits=mm  TranslationStandardAxis=+Z  TranslationCartesianOffset=[-25.865414462389737 -22.06740941499433 -1.136590821460004e-11]  TranslationCartesianOffsetUnits=mm  TranslationROffset=0  TranslationROffsetUnits=m  TranslationZOffset=0  TranslationZOffsetUnits=m  TranslationThetaOffset=0  TranslationThetaOffsetUnits=deg  RotationMethod=ArbitraryAxis  RotationAngleUnits=rad  RotationStandardAxis=+Z  RotationAngle=2.0943951023932001  RotationArbitraryAxis=[0 0 1]  FollAlignAxisA=+X  BaseAlignAxisA=+Y  FollAlignAxisB=+Y  BaseAlignAxisB=+Z  RotationSequenceAxes=FollowerAxes  RotationSequence=XYX  RotationSequenceAngles=[0 0 0]  RotationSequenceAnglesUnits=deg  RotationMatrix=[1 0 0; 0 1 0; 0 0 1]  Quaternion=[1 0 0 0]
  Transform5 : sm_lib/Frames and Transforms/Rigid Transform  TranslationMethod=Cartesian  TranslationStandardOffset=0  TranslationStandardOffsetUnits=mm  TranslationStandardAxis=+Z  TranslationCartesianOffset=[-25.86541446238942 -22.06740941499471 -1.136590821460004e-11]  TranslationCartesianOffsetUnits=mm  TranslationROffset=0  TranslationROffsetUnits=m  TranslationZOffset=0  TranslationZOffsetUnits=m  TranslationThetaOffset=0  TranslationThetaOffsetUnits=deg  RotationMethod=ArbitraryAxis  RotationAngleUnits=rad  RotationStandardAxis=+Z  RotationAngle=2.0943951023931855  RotationArbitraryAxis=[-0 -0 -1]  FollAlignAxisA=+X  BaseAlignAxisA=+Y  FollAlignAxisB=+Y  BaseAlignAxisB=+Z  RotationSequenceAxes=FollowerAxes  RotationSequence=XYX  RotationSequenceAngles=[0 0 0]  RotationSequenceAnglesUnits=deg  RotationMatrix=[1 0 0; 0 1 0; 0 0 1]  Quaternion=[1 0 0 0]
  Transform6 : sm_lib/Frames and Transforms/Rigid Transform  TranslationMethod=Cartesian  TranslationStandardOffset=0  TranslationStandardOffsetUnits=mm  TranslationStandardAxis=+Z  TranslationCartesianOffset=[-25.865414462390763 -22.06740941499276 9.9999999999886313]  TranslationCartesianOffsetUnits=mm  TranslationROffset=0  TranslationROffsetUnits=m  TranslationZOffset=0  TranslationZOffsetUnits=m  TranslationThetaOffset=0  TranslationThetaOffsetUnits=deg  RotationMethod=ArbitraryAxis  RotationAngleUnits=rad  RotationStandardAxis=+Z  RotationAngle=2.0943951023932006  RotationArbitraryAxis=[0 0 1]  FollAlignAxisA=+X  BaseAlignAxisA=+Y  FollAlignAxisB=+Y  BaseAlignAxisB=+Z  RotationSequenceAxes=FollowerAxes  RotationSequence=XYX  RotationSequenceAngles=[0 0 0]  RotationSequenceAnglesUnits=deg  RotationMatrix=[1 0 0; 0 1 0; 0 0 1]  Quaternion=[1 0 0 0]
  F : PMIOPort  Side=Right
  F3 : PMIOPort  Port=2  Side=Left
  F2 : PMIOPort  Port=3  Side=Right
  F1 : PMIOPort  Port=4  Side=Right
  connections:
  Transform/LConn1 -- Transform5/LConn1 -- Transform6/LConn1 -- Transform4/LConn1 -- ReferenceFrame/RConn1 -- F3/RConn1 -- Transform3/LConn1 -- Transform2/LConn1 -- Transform1/LConn1
  Transform/RConn1 -- F/RConn1
  Transform1/RConn1 -- F1/RConn1
  Transform2/RConn1 -- F2/RConn1
  BATI2_3_RIGID/LConn1 -- Transform3/RConn1
  BATI1_1_RIGID/LConn1 -- Transform4/RConn1
  BATI3_3_RIGID/LConn1 -- Transform5/RConn1
  PIED_1_RIGID/LConn1 -- Transform6/RConn1

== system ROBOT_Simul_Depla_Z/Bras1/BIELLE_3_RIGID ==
  ReferenceFrame : sm_lib/Frames and Transforms/Reference Frame
  Solid : sm_lib/Body Elements/File Solid  ExtGeomFileName=\STL\BIELLE_Défaut_sldprt.STL  UnitType=Custom  ExtGeomFileUnits=mm  StepReaderType=HEX  ExportConvexHullGeometry=off  InertiaType=Custom  Mass=0.008350539405564527  MassUnits=kg  CenterOfMass=[0 1.3968069938607398e-07 -5.4963035279888423e-06]  CenterOfMassUnits=mm  MomentsOfInertia=[9.7237898508136684 9.7147278737202658 0.035523108889582884]  MomentsOfInertiaUnits=kg*mm^2  ProductsOfInertia=[0 -4.4011490170351759e-08 -8.1673382975267321e-07]  ProductsOfInertiaUnits=kg*mm^2  BasedOnType=Density  Density=1000  DensityUnits=kg/(m^3)  DoExposeReferenceFrame=on  SerializedFrames=<Frames/>  GraphicType=FromGeometry  MarkerShape=Sphere  MarkerSize=10  MarkerSizeUnits=m  GraphicVisPropType=SimpleVisualProperties  GraphicDiffuseColor=[0.69803921568627447 0.69803921568627447 0.69803921568627447]  GraphicSpecularColor=[0.5 0.5 0.5 1.0]  GraphicAmbientColor=[0.15 0.15 0.15 1.0]  GraphicEmissiveColor=[0.0 0.0 0.0 1.0]  GraphicShininess=75  GraphicOpacity=1
  Transform : sm_lib/Frames and Transforms/Rigid Transform  TranslationMethod=Cartesian  TranslationStandardOffset=0  TranslationStandardOffsetUnits=mm  TranslationStandardAxis=+Z  TranslationCartesianOffset=[0 4.9999999999999902 -51.25]  TranslationCartesianOffsetUnits=mm  TranslationROffset=0  TranslationROffsetUnits=m  TranslationZOffset=0  TranslationZOffsetUnits=m  TranslationThetaOffset=0  TranslationThetaOffsetUnits=deg  RotationMethod=ArbitraryAxis  RotationAngleUnits=rad  RotationStandardAxis=+Z  RotationAngle=2.0943951023931957  RotationArbitraryAxis=[0.57735026918962584 -0.57735026918962573 0.57735026918962573]  FollAlignAxisA=+X  BaseAlignAxisA=+Y  FollAlignAxisB=+Y  BaseAlignAxisB=+Z  RotationSequenceAxes=FollowerAxes  RotationSequence=XYX  RotationSequenceAngles=[0 0 0]  RotationSequenceAnglesUnits=deg  RotationMatrix=[1 0 0; 0 1 0; 0 0 1]  Quaternion=[1 0 0 0]
  Transform1 : sm_lib/Frames and Transforms/Rigid Transform  TranslationMethod=Cartesian  TranslationStandardOffset=0  TranslationStandardOffsetUnits=mm  TranslationStandardAxis=+Z  TranslationCartesianOffset=[0 4.9999999999999769 51.249999999999986]  TranslationCartesianOffsetUnits=mm  TranslationROffset=0  TranslationROffsetUnits=m  TranslationZOffset=0  TranslationZOffsetUnits=m  TranslationThetaOffset=0  TranslationThetaOffsetUnits=deg  RotationMethod=ArbitraryAxis  RotationAngleUnits=rad  RotationStandardAxis=+Z  RotationAngle=2.0943951023931957  RotationArbitraryAxis=[0.57735026918962584 -0.57735026918962573 0.57735026918962573]  FollAlignAxisA=+X  BaseAlignAxisA=+Y  FollAlignAxisB=+Y  BaseAlignAxisB=+Z  RotationSequenceAxes=FollowerAxes  RotationSequence=XYX  RotationSequenceAngles=[0 0 0]  RotationSequenceAnglesUnits=deg  RotationMatrix=[1 0 0; 0 1 0; 0 0 1]  Quaternion=[1 0 0 0]
  F1 : PMIOPort  Side=Left
  F : PMIOPort  Port=2  Side=Right
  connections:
  Solid/RConn1 -- ReferenceFrame/RConn1 -- Transform/LConn1 -- Transform1/LConn1
  Transform/RConn1 -- F/RConn1
  Transform1/RConn1 -- F1/RConn1

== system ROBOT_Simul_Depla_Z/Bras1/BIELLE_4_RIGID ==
  ReferenceFrame : sm_lib/Frames and Transforms/Reference Frame
  Solid : sm_lib/Body Elements/File Solid  ExtGeomFileName=\STL\BIELLE_Défaut_sldprt.STL  UnitType=Custom  ExtGeomFileUnits=mm  StepReaderType=HEX  ExportConvexHullGeometry=off  InertiaType=Custom  Mass=0.008350539405564527  MassUnits=kg  CenterOfMass=[0 1.3968069938607398e-07 -5.4963035279888423e-06]  CenterOfMassUnits=mm  MomentsOfInertia=[9.7237898508136684 9.7147278737202658 0.035523108889582884]  MomentsOfInertiaUnits=kg*mm^2  ProductsOfInertia=[0 -4.4011490170351759e-08 -8.1673382975267321e-07]  ProductsOfInertiaUnits=kg*mm^2  BasedOnType=Density  Density=1000  DensityUnits=kg/(m^3)  DoExposeReferenceFrame=on  SerializedFrames=<Frames/>  GraphicType=FromGeometry  MarkerShape=Sphere  MarkerSize=10  MarkerSizeUnits=m  GraphicVisPropType=SimpleVisualProperties  GraphicDiffuseColor=[0.69803921568627447 0.69803921568627447 0.69803921568627447]  GraphicSpecularColor=[0.5 0.5 0.5 1.0]  GraphicAmbientColor=[0.15 0.15 0.15 1.0]  GraphicEmissiveColor=[0.0 0.0 0.0 1.0]  GraphicShininess=75  GraphicOpacity=1
  Transform : sm_lib/Frames and Transforms/Rigid Transform  TranslationMethod=Cartesian  TranslationStandardOffset=0  TranslationStandardOffsetUnits=mm  TranslationStandardAxis=+Z  TranslationCartesianOffset=[0 4.9999999999999902 -51.250000000000014]  TranslationCartesianOffsetUnits=mm  TranslationROffset=0  TranslationROffsetUnits=m  TranslationZOffset=0  TranslationZOffsetUnits=m  TranslationThetaOffset=0  TranslationThetaOffsetUnits=deg  RotationMethod=ArbitraryAxis  RotationAngleUnits=rad  RotationStandardAxis=+Z  RotationAngle=2.0943951023931953  RotationArbitraryAxis=[0.57735026918962584 -0.57735026918962584 0.57735026918962584]  FollAlignAxisA=+X  BaseAlignAxisA=+Y  FollAlignAxisB=+Y  BaseAlignAxisB=+Z  RotationSequenceAxes=FollowerAxes  RotationSequence=XYX  RotationSequenceAngles=[0 0 0]  RotationSequenceAnglesUnits=deg  RotationMatrix=[1 0 0; 0 1 0; 0 0 1]  Quaternion=[1 0 0 0]
  Transform1 : sm_lib/Frames and Transforms/Rigid Transform  TranslationMethod=Cartesian  TranslationStandardOffset=0  TranslationStandardOffsetUnits=mm  TranslationStandardAxis=+Z  TranslationCartesianOffset=[0 5.0000000000000044 51.250000000000014]  TranslationCartesianOffsetUnits=mm  TranslationROffset=0  TranslationROffsetUnits=m  TranslationZOffset=0  TranslationZOffsetUnits=m  TranslationThetaOffset=0  TranslationThetaOffsetUnits=deg  RotationMethod=ArbitraryAxis  RotationAngleUnits=rad  RotationStandardAxis=+Z  RotationAngle=2.0943951023931953  RotationArbitraryAxis=[0.57735026918962584 -0.57735026918962584 0.57735026918962584]  FollAlignAxisA=+X  BaseAlignAxisA=+Y  FollAlignAxisB=+Y  BaseAlignAxisB=+Z  RotationSequenceAxes=FollowerAxes  RotationSequence=XYX  RotationSequenceAngles=[0 0 0]  RotationSequenceAnglesUnits=deg  RotationMatrix=[1 0 0; 0 1 0; 0 0 1]  Quaternion=[1 0 0 0]
  F1 : PMIOPort  Side=Left
  F : PMIOPort  Port=2  Side=Right
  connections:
  Solid/RConn1 -- ReferenceFrame/RConn1 -- Transform/LConn1 -- Transform1/LConn1
  Transform/RConn1 -- F/RConn1
  Transform1/RConn1 -- F1/RConn1

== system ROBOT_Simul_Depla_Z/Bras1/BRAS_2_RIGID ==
  BRAS_1_RIGID : Subsystem
  BRAS_3_RIGID : Subsystem
  ReferenceFrame : sm_lib/Frames and Transforms/Reference Frame
  Transform : sm_lib/Frames and Transforms/Rigid Transform  TranslationMethod=Cartesian  TranslationStandardOffset=0  TranslationStandardOffsetUnits=mm  TranslationStandardAxis=+Z  TranslationCartesianOffset=[-9.6989083431253675e-13 -16.842456388464441 -5.0000000000000027]  TranslationCartesianOffsetUnits=mm  TranslationROffset=0  TranslationROffsetUnits=m  TranslationZOffset=0  TranslationZOffsetUnits=m  TranslationThetaOffset=0  TranslationThetaOffsetUnits=deg  RotationMethod=ArbitraryAxis  RotationAngleUnits=rad  RotationStandardAxis=+Z  RotationAngle=1.852259063952334e-15  RotationArbitraryAxis=[-0.27659366947124742 0.96098696245497017 -2.4616792487648572e-16]  FollAlignAxisA=+X  BaseAlignAxisA=+Y  FollAlignAxisB=+Y  BaseAlignAxisB=+Z  RotationSequenceAxes=FollowerAxes  RotationSequence=XYX  RotationSequenceAngles=[0 0 0]  RotationSequenceAnglesUnits=deg  RotationMatrix=[1 0 0; 0 1 0; 0 0 1]  Quaternion=[1 0 0 0]
  Transform1 : sm_lib/Frames and Transforms/Rigid Transform  TranslationMethod=Cartesian  TranslationStandardOffset=0  TranslationStandardOffsetUnits=mm  TranslationStandardAxis=+Z  TranslationCartesianOffset=[0 43.157543611535324 10.000000000006278]  TranslationCartesianOffsetUnits=mm  TranslationROffset=0  TranslationROffsetUnits=m  TranslationZOffset=0  TranslationZOffsetUnits=m  TranslationThetaOffset=0  TranslationThetaOffsetUnits=deg  RotationMethod=ArbitraryAxis  RotationAngleUnits=rad  RotationStandardAxis=+Z  RotationAngle=3.1415926535897931  RotationArbitraryAxis=[1 0 0]  FollAlignAxisA=+X  BaseAlignAxisA=+Y  FollAlignAxisB=+Y  BaseAlignAxisB=+Z  RotationSequenceAxes=FollowerAxes  RotationSequence=XYX  RotationSequenceAngles=[0 0 0]  RotationSequenceAnglesUnits=deg  RotationMatrix=[1 0 0; 0 1 0; 0 0 1]  Quaternion=[1 0 0 0]
  Transform2 : sm_lib/Frames and Transforms/Rigid Transform  TranslationMethod=Cartesian  TranslationStandardOffset=0  TranslationStandardOffsetUnits=mm  TranslationStandardAxis=+Z  TranslationCartesianOffset=[0 -16.842456388464662 6.2727600891321345e-12]  TranslationCartesianOffsetUnits=mm  TranslationROffset=0  TranslationROffsetUnits=m  TranslationZOffset=0  TranslationZOffsetUnits=m  TranslationThetaOffset=0  TranslationThetaOffsetUnits=deg  RotationMethod=None  RotationAngleUnits=deg  RotationStandardAxis=+Z  RotationAngle=0  RotationArbitraryAxis=[0 0 1]  FollAlignAxisA=+X  BaseAlignAxisA=+Y  FollAlignAxisB=+Y  BaseAlignAxisB=+Z  RotationSequenceAxes=FollowerAxes  RotationSequence=XYX  RotationSequenceAngles=[0 0 0]  RotationSequenceAnglesUnits=deg  RotationMatrix=[1 0 0; 0 1 0; 0 0 1]  Quaternion=[1 0 0 0]
  Transform3 : sm_lib/Frames and Transforms/Rigid Transform  TranslationMethod=Cartesian  TranslationStandardOffset=0  TranslationStandardOffsetUnits=mm  TranslationStandardAxis=+Z  TranslationCartesianOffset=[0 43.157543611535324 6.2796989830360417e-12]  TranslationCartesianOffsetUnits=mm  TranslationROffset=0  TranslationROffsetUnits=m  TranslationZOffset=0  TranslationZOffsetUnits=m  TranslationThetaOffset=0  TranslationThetaOffsetUnits=deg  RotationMethod=ArbitraryAxis  RotationAngleUnits=rad  RotationStandardAxis=+Z  RotationAngle=3.1415926535897931  RotationArbitraryAxis=[0 0 1]  FollAlignAxisA=+X  BaseAlignAxisA=+Y  FollAlignAxisB=+Y  BaseAlignAxisB=+Z  RotationSequenceAxes=FollowerAxes  RotationSequence=XYX  RotationSequenceAngles=[0 0 0]  RotationSequenceAnglesUnits=deg  RotationMatrix=[1 0 0; 0 1 0; 0 0 1]  Quaternion=[1 0 0 0]
  F : PMIOPort  Side=Left
  F1 : PMIOPort  Port=2  Side=Right
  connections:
  Transform/LConn1 -- ReferenceFrame/RConn1 -- Transform1/LConn1 -- Transform2/LConn1 -- Transform3/LConn1
  Transform/RConn1 -- F/RConn1
  Transform1/RConn1 -- F1/RConn1
  BRAS_1_RIGID/LConn1 -- Transform2/RConn1
  BRAS_3_RIGID/LConn1 -- Transform3/RConn1
